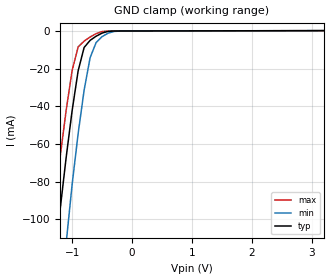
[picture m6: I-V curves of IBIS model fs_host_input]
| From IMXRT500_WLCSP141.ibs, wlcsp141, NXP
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[Model] fs_host_input
|   Model fs_host_input
| Library cells for typ/min/max conditions are connected as defined below:
|  pad_usbdp - External Pad
|  d_dmpulldn - vddd
|  d_dppulldn - vddd
|  d_sw1_neg - gnda
|  d_sw1_pos - gnda
|  d_sw2_neg - gnda
|  d_sw2_pos - gnda
|  gnda - gnda
|  pad_usb_vss - pad_usb_vss
|  usb2_reg_tx_fs_hiz - vddd
|  usb2_reg_tx_hs_term - gnda
|  usb2_reg_tx_hs_xcvr - gnda
|  usb2_reg_tx_ls_en - gnda
|  usbphy_d2a_txhsactive - gnda
|  vddb - vddb
|  vddd - vddd
| All other pins connected to ground
Model_type Input
Vinl =   0.800V
Vinh =   2.000V
C_comp   2.8431pF   2.6338pF   3.0727pF
[Temperature Range]   27.0000   0.1250k   -40.0000
[Voltage Range]   3.1500V   3.0000V   3.3000V
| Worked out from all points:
|   GND clamp passes 1 mA (typ) near -0.49 V on its own axis
[GND_clamp]
|Voltage   I(typ)   I(min)   I(max)
-3.3V     -1.77A     -1.861A    -1.685A
-1.4V     -157.5mA   -242mA     -123.3mA
-1.3V     -124.5mA   -192.1mA   -93.95mA
-1.2V     -94.77mA   -149.4mA   -66.85mA
-1.1V     -67.27mA   -112.8mA   -42.22mA
-1V       -42.3mA    -81.55mA   -20.98mA
-900mV    -21.24mA   -54.58mA   -8.478mA
-800mV    -8.783mA   -31.46mA   -5.373mA
-700mV    -5.002mA   -14.24mA   -3.221mA
-600mV    -2.797mA   -6.151mA   -1.432mA
-200mV    -10.86uA   -44.63uA   -10.07uA
3.2V      168uA      211.3uA    161.1uA
